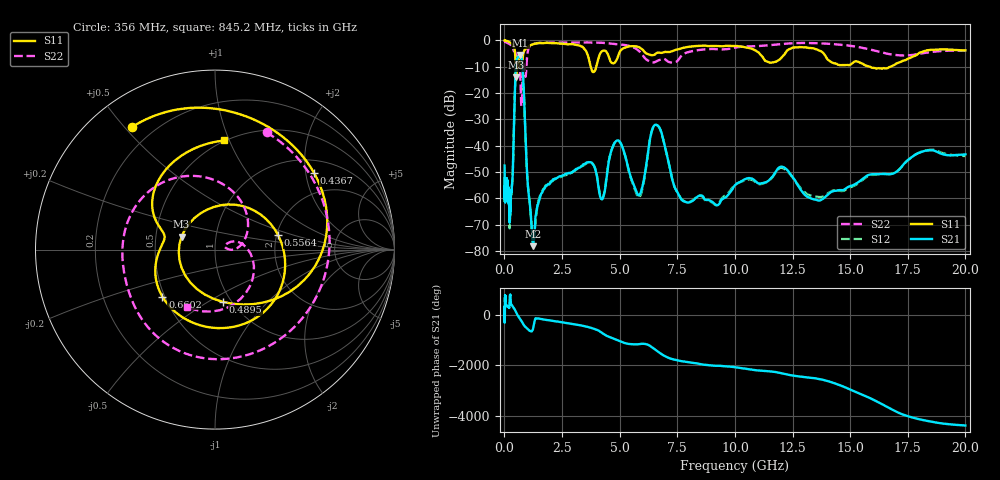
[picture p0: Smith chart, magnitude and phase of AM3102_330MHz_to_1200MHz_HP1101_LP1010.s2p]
! Date/Time: Tue, Sep 11, 2018 5:22 PM
! Network Analyzer: Agilent Technologies E8362B Rev: A.07.50.63
! Sweep from 0.010 to 20.000 GHz, 1601 Points, Sweep Type: LOG
! Power Supply: 4.949 V, 0.001 A
# Hz S DB R 50
!freq MagS11 AngS11 MagS21 AngS21 MagS12 AngS12 MagS22 AngS22
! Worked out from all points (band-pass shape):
!   1601 points, 10 MHz to 20 GHz, reference 50 ohm
!   highest |S21| = -5.52 dB at 689.1 MHz (marker M1); lowest = -78.2 dB at 1.242 GHz (marker M2)
!   |S21| within 3 dB of the highest: 510.3 MHz to 772.4 MHz (262.1 MHz wide, 40.9 % of centre)
!   lowest |S11| = -14.0 dB at 513.3 MHz (marker M3), VSWR 1.50, Z = 34 + j5.1 ohm
!   |S11| at or under -10 dB: 487.3 MHz to 544.9 MHz (57.56 MHz wide, 11.2 % of centre); 3.747 GHz to 3.985 GHz (238.7 MHz wide, 6.17 % of centre); 15.86 GHz to 16.74 GHz (886.5 MHz wide, 5.44 % of centre)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
!   |S22| runs from -25.0 to -0.2 dB; largest |S21 - S12| = 0.0087
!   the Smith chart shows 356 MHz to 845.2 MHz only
!   S11 on the Smith chart (normalised r, x): 356 MHz: 0.12, +0.52; 436.7 MHz: 1.34, +2.23; 489.5 MHz: 0.91, -0.58; 556.4 MHz: 2.03, +0.39; 660.2 MHz: 0.49, -0.30; 845.2 MHz: 0.49, +0.96
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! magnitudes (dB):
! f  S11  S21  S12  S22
! 10 MHz  0.0  -47.6  -53.1  -0.2
! 35.55 MHz  -0.1  -60.6  -57.5  -0.4
! 126.4 MHz  -0.2  -53.5  -54.1  -0.9
! 232.2 MHz  -0.7  -68.4  -70.1  -1.4
! 356 MHz  -1.7  -52.1  -52.2  -2.9
! 436.7 MHz  -3.1  -25.5  -25.5  -4.2
! 447.2 MHz  -3.6  -22.2  -22.2  -4.2
! 489.5 MHz  -10.6  -11.4  -11.4  -4.9
! 513.3 MHz  -14.0  -8.3  -8.4  -5.5
! 556.4 MHz  -8.9  -6.8  -6.8  -5.8
! 660.2 MHz  -8.1  -5.6  -5.7  -9.9
! 689.1 MHz  -9.4  -5.5  -5.6  -13.5
! 845.2 MHz  -4.3  -19.7  -19.8  -9.0
! 1.242 GHz  -1.5  -78.2  -76.5  -1.3
! 1.59 GHz  -1.0  -58.3  -58.0  -0.9
! 3.668 GHz  -7.2  -46.2  -46.1  -0.8
! 4.23 GHz  -4.2  -60.4  -60.0  -0.9
! 4.902 GHz  -6.8  -38.0  -38.1  -1.5
! 5.652 GHz  -2.2  -55.8  -56.3  -2.9
! 6.58 GHz  -4.9  -32.1  -32.1  -8.0
! 7.92 GHz  -2.5  -61.6  -61.3  -4.6
! 20 GHz  -3.8  -43.3  -43.9  -3.9
